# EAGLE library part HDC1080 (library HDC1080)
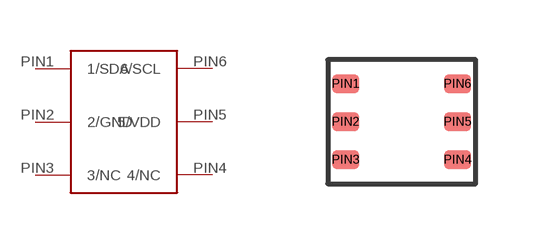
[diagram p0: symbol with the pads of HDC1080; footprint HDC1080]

Designator prefix -

## HDC1080  [HDC1080]
PIN1  1/SDA
PIN2  2/GND
PIN3  3/NC
PIN4  4/NC
PIN5  5/VDD
PIN6  6/SCL

## Footprint HDC1080 (pad centres in mm)
smd 0.67 x 0.47: PIN1 -1.4,0.95; PIN2 -1.4,0; PIN3 -1.4,-0.95; PIN4 1.4,-0.95; PIN5 1.4,0; PIN6 1.4,0.95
